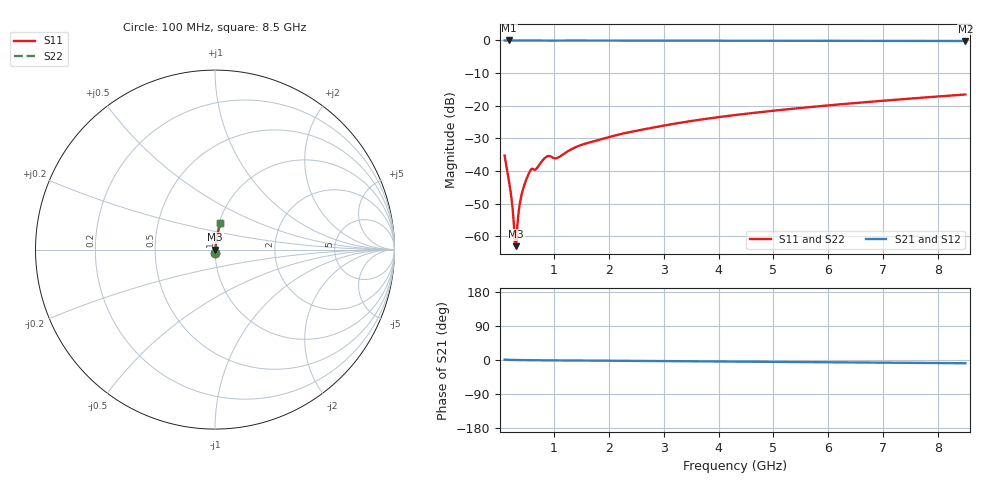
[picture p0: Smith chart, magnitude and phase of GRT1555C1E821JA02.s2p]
!Murata Part Number: GRT1555C1E821JA02
!These Parameters are Measured in Series Mode Connection
!Data Generated on Jun 19, 2026
!  o--ll--o
!Port1  Port2
!  o------o
!Operation Temp=25[degC], DC Bias Voltage=0[V]
!Freq. Start=100[MHz] Stop=9[GHz] 401[Steps]
# Hz S RI R 50
!Freq.(Hz) S11(Real) S11(Imag) S21(Real) S21(Imag) S12(Real) S12(Imag) S22(Real) S22(Imag)
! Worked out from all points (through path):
!   401 points, 100 MHz to 8.5 GHz, reference 50 ohm
!   highest |S21| = 0.00 dB at 184 MHz (marker M1); lowest = -0.2 dB at 8.5 GHz (marker M2)
!   group delay of S21, straight-line fit = 2.8 ps
!   lowest |S11| = -63.0 dB at 310 MHz (marker M3), VSWR 1.00, Z = 50.1 + j0.043 ohm
!   |S11| at or under -10 dB: start of sweep to end of sweep
!   |S22| runs from -63.0 to -16.5 dB; largest |S21 - S12| = 0
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1e8  0.000713 -0.0173  0.9993 0.0173  0.9993 0.0173  0.000713 -0.0173
1.42e8  0.000543 -0.0106  0.9995 0.0106  0.9995 0.0106  0.000543 -0.0106
1.84e8  0.000495 -0.00662  0.9995 0.00662  0.9995 0.00662  0.000495 -0.00662
2.26e8  0.000493 -0.00376  0.9995 0.00376  0.9995 0.00376  0.000493 -0.00376
2.68e8  0.000518 -0.00149  0.9995 0.00149  0.9995 0.00149  0.000518 -0.00149
2.89e8  0.000538 -0.000496  0.9995 0.000496  0.9995 0.000496  0.000538 -0.000496
3.1e8  0.000564 0.000429  0.9994 -0.000429  0.9994 -0.000429  0.000564 0.000429
3.31e8  0.000594 0.0013  0.9994 -0.0013  0.9994 -0.0013  0.000594 0.0013
3.73e8  0.000674 0.00294  0.9993 -0.00294  0.9993 -0.00294  0.000674 0.00294
4.15e8  0.000788 0.00447  0.9992 -0.00447  0.9992 -0.00447  0.000788 0.00447
4.78e8  0.00108 0.00672  0.9989 -0.00672  0.9989 -0.00672  0.00108 0.00672
5.62e8  0.00226 0.00968  0.9977 -0.00968  0.9977 -0.00968  0.00226 0.00968
6.88e8  0.00283 0.0107  0.9972 -0.0107  0.9972 -0.0107  0.00283 0.0107
8.77e8  0.00552 0.0159  0.9945 -0.0159  0.9945 -0.0159  0.00552 0.0159
1.066e9  0.00472 0.0152  0.9953 -0.0152  0.9953 -0.0152  0.00472 0.0152
1.507e9  0.00461 0.0249  0.9954 -0.0249  0.9954 -0.0249  0.00461 0.0249
2.221e9  0.00576 0.0365  0.9942 -0.0365  0.9942 -0.0365  0.00576 0.0365
2.914e9  0.00681 0.0477  0.9932 -0.0477  0.9932 -0.0477  0.00681 0.0477
4.3e9  0.0107 0.0712  0.9893 -0.0712  0.9893 -0.0712  0.0107 0.0712
5.707e9  0.016 0.0948  0.984 -0.0948  0.984 -0.0948  0.016 0.0948
7.114e9  0.0223 0.1194  0.9777 -0.1194  0.9777 -0.1194  0.0223 0.1194
8.5e9  0.0302 0.1458  0.9698 -0.1458  0.9698 -0.1458  0.0302 0.1458
